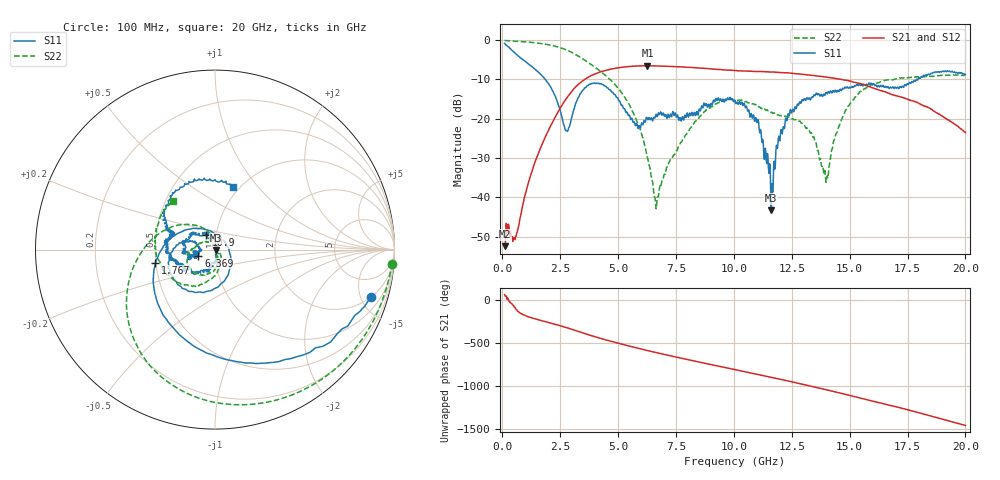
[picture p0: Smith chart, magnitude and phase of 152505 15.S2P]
!  2-Port S-parameters saved by WinCal
! VAR MeasName=S-Parameters (CALIBRATED_DATA) read from VNA (N5230C)
! VAR MeasDate=4/10/2015 9:29:46 AM
! VAR NAME=152505 15
! VAR FILENAME=152505 15.S2P
! VAR DATE=4/10/2015 9:29:46 AM
! VAR PHYS_PORTS=1,2
# Hz S DB R 50
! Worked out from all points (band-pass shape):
!   801 points, 100 MHz to 20 GHz, reference 50 ohm
!   highest |S21| = -6.53 dB at 6.269 GHz (marker M1); lowest = -52.4 dB at 100 MHz (marker M2)
!   |S21| within 3 dB of the highest: 3.68 GHz to 14.15 GHz (10.46 GHz wide, 117 % of centre)
!   lowest |S11| = -43.3 dB at 11.62 GHz (marker M3), VSWR 1.01, Z = 50.6 - j0.25 ohm
!   |S11| at or under -10 dB: 1.853 GHz to 17.88 GHz (16.03 GHz wide, 162 % of centre); 17.89594 GHz to 17.95168 GHz (55.74 MHz wide, 0.311 % of centre)
!   |S22| runs from -42.9 to -0.1 dB; largest |S21 - S12| = 0.0077
!   S11 on the Smith chart (normalised r, x): 100 MHz: 2.03, -6.06; 1.767 GHz: 0.50, -0.08; 6.369 GHz: 0.83, -0.06; 10.9 GHz: 0.90, +0.14; 20 GHz: 0.93, +0.75
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1e8  -0.85 -16.9  -52.43 58.5  -52.56 58.4  -0.09 -4.5
6.4725e8  -3.82 -77.0  -48.76 -129.4  -48.81 -128.4  -0.31 -26.3
1.1945e9  -6.33 -122.4  -34.93 153.5  -34.97 153.7  -0.55 -48.3
1.766625e9  -9.38 -167.5  -25.84 110.5  -25.85 110.5  -0.95 -72.1
2.7865e9  -23.06 36.4  -14.71 32.3  -14.71 32.6  -2.53 -118.0
3.43325e9  -13.11 -92.4  -10.55 -24.5  -10.51 -24.2  -4.61 -146.9
4.552625e9  -12.16 -175.7  -7.58 -115.0  -7.58 -115.0  -9.46 166.7
5.42325e9  -18.92 161.9  -6.74 -176.5  -6.73 -176.6  -15.87 125.9
6.269e9  -20.15 -162.1  -6.53 127.2  -6.55 127.0  -29.85 81.9
6.3685e9  -20.20 -160.3  -6.54 120.9  -6.57 120.8  -32.36 74.9
6.741625e9  -18.49 -169.4  -6.59 97.8  -6.57 97.4  -39.90 -55.1
8.30875e9  -18.37 -157.2  -7.03 4.3  -7.04 4.4  -20.79 -83.5
1.005e10  -15.30 161.1  -7.73 -94.7  -7.77 -94.9  -15.30 -144.8
1.089575e10  -20.64 121.0  -7.96 -142.0  -7.98 -142.1  -16.43 -170.8
1.161712e10  -43.33 -21.3  -8.11 176.1  -8.11 175.8  -18.34 176.5
1.23385e10  -18.73 -105.5  -8.33 132.8  -8.36 132.4  -19.49 170.3
1.338325e10  -14.53 -142.6  -8.98 69.3  -8.90 69.3  -24.21 137.1
1.398025e10  -13.26 -156.0  -9.38 31.8  -9.31 31.4  -36.19 40.2
1.49255e10  -12.09 -166.7  -10.30 -29.7  -10.43 -30.5  -16.86 -89.3
1.669162e10  -12.23 161.1  -13.50 -147.0  -13.57 -147.8  -10.12 -160.4
1.815925e10  -9.24 144.8  -16.63 111.3  -16.55 111.9  -9.31 164.9
2e10  -8.76 74.0  -23.51 -24.3  -23.52 -23.7  -8.99 131.0
